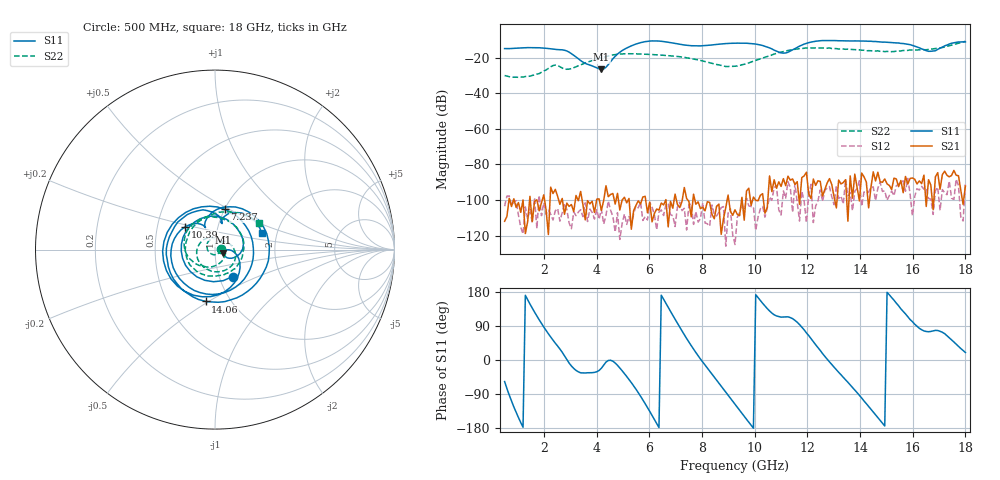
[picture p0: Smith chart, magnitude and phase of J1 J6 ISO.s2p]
!Agilent Technologies,N5230A,MY45001360,A.07.50.67
!Agilent N5230A: A.07.50.67
!Date: Tuesday, April 16, 2024 16:33:08
!Correction: S11(Full 2 Port(1,2))
!S21(Full 2 Port(1,2))
!S12(Full 2 Port(1,2))
!S22(Full 2 Port(1,2))
!S2P File: Measurements: S11, S21, S12, S22:
# Hz S  dB  R 50
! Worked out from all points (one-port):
!   201 points, 500 MHz to 18 GHz, reference 50 ohm
!   lowest |S11| = -26.6 dB at 4.175 GHz (marker M1), VSWR 1.10, Z = 54.5 - j1.9 ohm
!   |S11| at or under -10 dB: start of sweep to end of sweep
!   S11 on the Smith chart (normalised r, x): 500 MHz: 1.16, -0.36; 7.237 GHz: 1.00, +0.47; 10.39 GHz: 0.70, +0.18; 14.06 GHz: 0.77, -0.48; 18 GHz: 1.66, +0.34
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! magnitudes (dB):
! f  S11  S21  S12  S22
! 500 MHz  -14.9  -111.9  -103.5  -30.1
! 1.462 GHz  -14.4  -97.9  -105.1  -30.4
! 2.337 GHz  -15.2  -96.3  -111.2  -24.5
! 2.688 GHz  -15.6  -99.1  -107.1  -25.9
! 3.038 GHz  -17.8  -102.5  -116.1  -26.2
! 3.475 GHz  -22.5  -102.6  -109.3  -23.6
! 4.175 GHz  -26.6  -105.9  -105.2  -20.1
! 5.138 GHz  -14.6  -101.6  -113.7  -17.8
! 5.75 GHz  -11.3  -98.3  -111.5  -18.0
! 6.362 GHz  -10.7  -105.7  -106.8  -18.5
! 7.237 GHz  -12.7  -100.8  -106.0  -19.7
! 8.9 GHz  -12.1  -104.2  -125.9  -25.0
! 9.25 GHz  -11.9  -105.5  -125.0  -24.8
! 10.39 GHz  -13.6  -107.4  -109.6  -19.7
! 11.18 GHz  -17.4  -91.9  -99.0  -16.3
! 12.22 GHz  -11.0  -88.2  -112.7  -14.6
! 14.06 GHz  -10.6  -84.9  -103.5  -15.8
! 15.11 GHz  -11.5  -91.8  -97.4  -16.7
! 15.9 GHz  -12.7  -87.8  -96.7  -15.7
! 16.6 GHz  -16.5  -88.6  -99.1  -15.4
! 17.48 GHz  -11.9  -86.2  -99.0  -12.9
! 18 GHz  -11.2  -92.1  -90.3  -10.8
